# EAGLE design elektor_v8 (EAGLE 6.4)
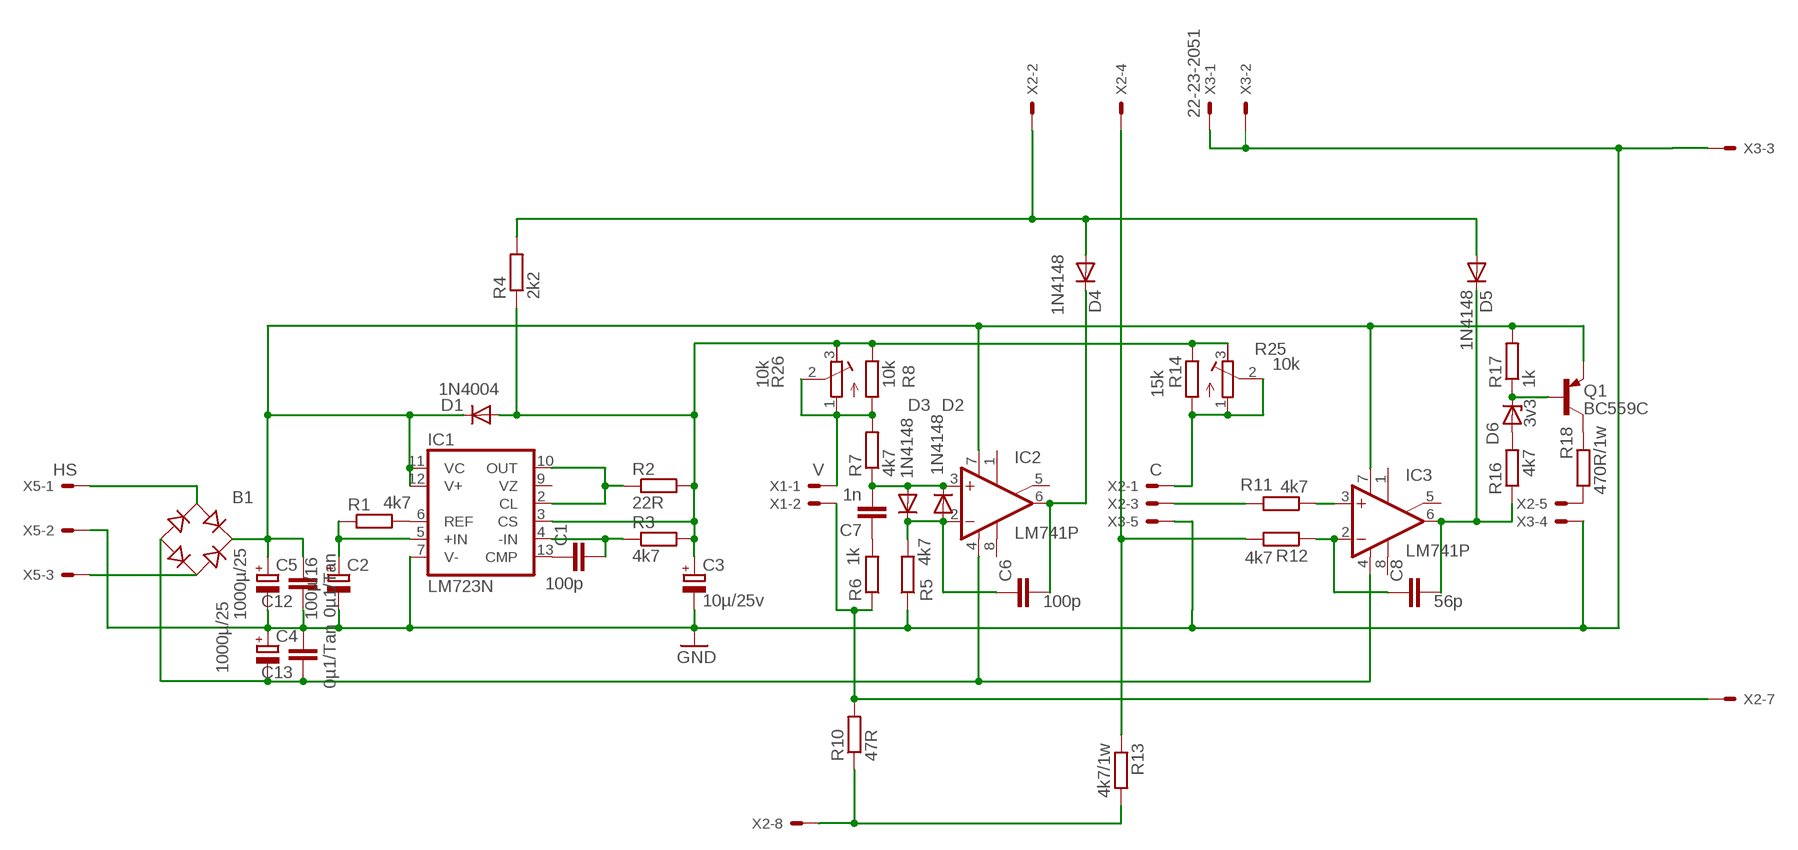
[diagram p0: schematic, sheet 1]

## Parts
B1  RB1A  [RB1A]
C1  100p  C-EU025-024X044  [C025-024X044]
C2  100µ/16  CPOL-EUE2.5-6  [E2,5-6]
C3  10µ/25v  CPOL-EUE2.5-6  [E2,5-6]
C4  1000µ/25  CPOL-EUE5-13  [E5-13]
C5  1000µ/25  CPOL-EUE5-13  [E5-13]
C6  100p  C-EU050-024X044  [C050-024X044]
C7  1n  C-EU050-024X044  [C050-024X044]
C8  56p  C-EU050-024X044  [C050-024X044]
C12  0µ1/Tan  C-EU025-024X044  [C025-024X044]
C13  0µ1/Tan  C-EU025-024X044  [C025-024X044]
D1  1N4004  [DO41-10]
D2  1N4148  1N4148DO35-7  [DO35-7]
D3  1N4148  1N4148DO35-7  [DO35-7]
D4  1N4148  1N4148DO35-7  [DO35-7]
D5  1N4148  1N4148DO35-7  [DO35-7]
D6  3v3  ZENER-DIODEDO34-7  [DO34Z7]
IC1  LM723N  [DIL14]
IC2  LM741P  [DIL08]
IC3  LM741P  [DIL08]
Q1  BC559C  [TO92-EBC]
R1  4k7  R-EU_0207/2V  [0207/2V]
R2  22R  R-EU_0207/2V  [0207/2V]
R3  4k7  R-EU_0207/2V  [0207/2V]
R4  2k2  R-EU_0204/7  [0204/7]
R5  4k7  R-EU_0207/2V  [0207/2V]
R6  1k  R-EU_0204/7  [0204/7]
R7  4k7  R-EU_0207/5V  [0207/5V]
R8  10k  R-EU_0207/2V  [0207/2V]
R10  47R  R-EU_0207/2V  [0207/2V]
R11  4k7  R-EU_0207/12  [0207/12]
R12  4k7  R-EU_0204/7  [0204/7]
R13  4k7/1w  R-EU_0204/7  [0204/7]
R14  15k  R-EU_0207/2V  [0207/2V]
R16  4k7  R-EU_0207/5V  [0207/5V]
R17  1k  R-EU_0207/5V  [0207/5V]
R18  470R/1w  R-EU_0204/7  [0204/7]
R25  10k  R-TRIMM64Y  [RTRIM64Y]
R26  10k  R-TRIMM64Y  [RTRIM64Y]
X1  V  22-23-2021  [22-23-2021]
X2  C  22-23-2081  [22-23-2081]
X3  22-23-2051  [22-23-2051]
X5  HS  22-23-2031  [22-23-2031]

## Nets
GND: C2.- C3.- C4.+ C5.- C12.1 C13.2 IC1.7(V-) R5.1 X3.1 X3.2 X3.3 X3.4 X3.5 X5.2
N$1: IC1.6(REF) R1.2
N$2: C2.+ IC1.5(+IN) R1.1
N$3: C1.1 IC1.13(CMP)
N$4: C1.2 IC1.4(-IN) R3.1
N$5: IC1.2(CL) IC1.10(OUT) R2.1
N$6: R12.2 R13.1 X2.4
N$7: C6.1 D2.A D3.C IC2.2(-IN) R5.2
N$8: R18.1 X2.5
N$9: C7.2 D2.C D3.A IC2.3(+IN) R7.1
N$10: C6.2 D4.C IC2.6(OUT)
N$11: R10.1 R13.2 X2.8
N$12: B1.AC1 X5.1
N$13: B1.AC2 X5.3
N$14: B1.+ C5.+ C12.2 D1.C IC1.11(VC) IC1.12(V+) IC2.7(V+) IC3.7(V+) Q1.E R17.2
N$15: B1.- C4.- C13.1 IC2.4(V-) IC3.4(V-)
N$16: C7.1 R6.2
N$17: R7.2 R8.1 R26.1(A) R26.2(S) X1.1
N$18: C3.+ D1.A IC1.3(CS) R2.2 R3.2 R4.1 R8.2 R14.2 R25.3(E) R26.3(E)
N$19: R6.1 R10.2 X1.2 X2.7
N$21: C8.2 D5.C IC3.6(OUT) R16.1
N$22: C8.1 IC3.2(-IN) R12.1
N$25: R11.2 X2.3
N$26: R14.1 R25.1(A) R25.2(S) X2.1
N$28: IC3.3(+IN) R11.1
N$29: D6.A R16.2
N$30: D6.C Q1.B R17.1
N$31: Q1.C R18.2
N$34: D4.A D5.A R4.2 X2.2
Unconnected: IC1.9(VZ) IC2.1(ON1) IC2.5(ON2) IC2.8(OPT) IC3.1(ON1) IC3.5(ON2) IC3.8(OPT) X2.6

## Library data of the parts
B1 = rectifier:RB1A: RECTIFIER 1 A
C1 C6-C8 C12 C13 = rcl:C-EU: CAPACITOR, European symbol
C2-C5 = rcl:CPOL-EU: POLARIZED CAPACITOR, European symbol
D1 = diode:1N4004: DIODE
D2-D5 = diode:1N4148: DIODE
D6 = diode:ZENER-DIODE: Z-Diode
IC1 = linear:*723: Positive VOLTAGE REGULATOR
IC2 IC3 = linear:*741: OP AMP
Q1 = transistor-pnp:BC559*: PNP Transistror
R1-R8 R10-R14 R16-R18 = rcl:R-EU_: RESISTOR, European symbol
R25 R26 = rcl:R-TRIMM: Trimm resistor
X1 = con-molex:22-23-2021: .100" (2.54mm) Center Header - 2 Pin; MF: MOLEX; MPN: 22-23-2021; OC_FARNELL: 1462926; OC_NEWARK: 25C3832
X2 = con-molex:22-23-2081: .100" (2.54mm) Center Header - 8 Pin; MF: MOLEX; MPN: 22-23-2081; OC_FARNELL: 1756826; OC_NEWARK: 01C7592
X3 = con-molex:22-23-2051: .100" (2.54mm) Center Header - 5 Pin; MF: MOLEX; MPN: 22-23-2051; OC_FARNELL: 1462952; OC_NEWARK: 38C9178
X5 = con-molex:22-23-2031: .100" (2.54mm) Center Header - 3 Pin; MF: MOLEX; MPN: 22-23-2031; OC_FARNELL: 1462950; OC_NEWARK: 30C0862

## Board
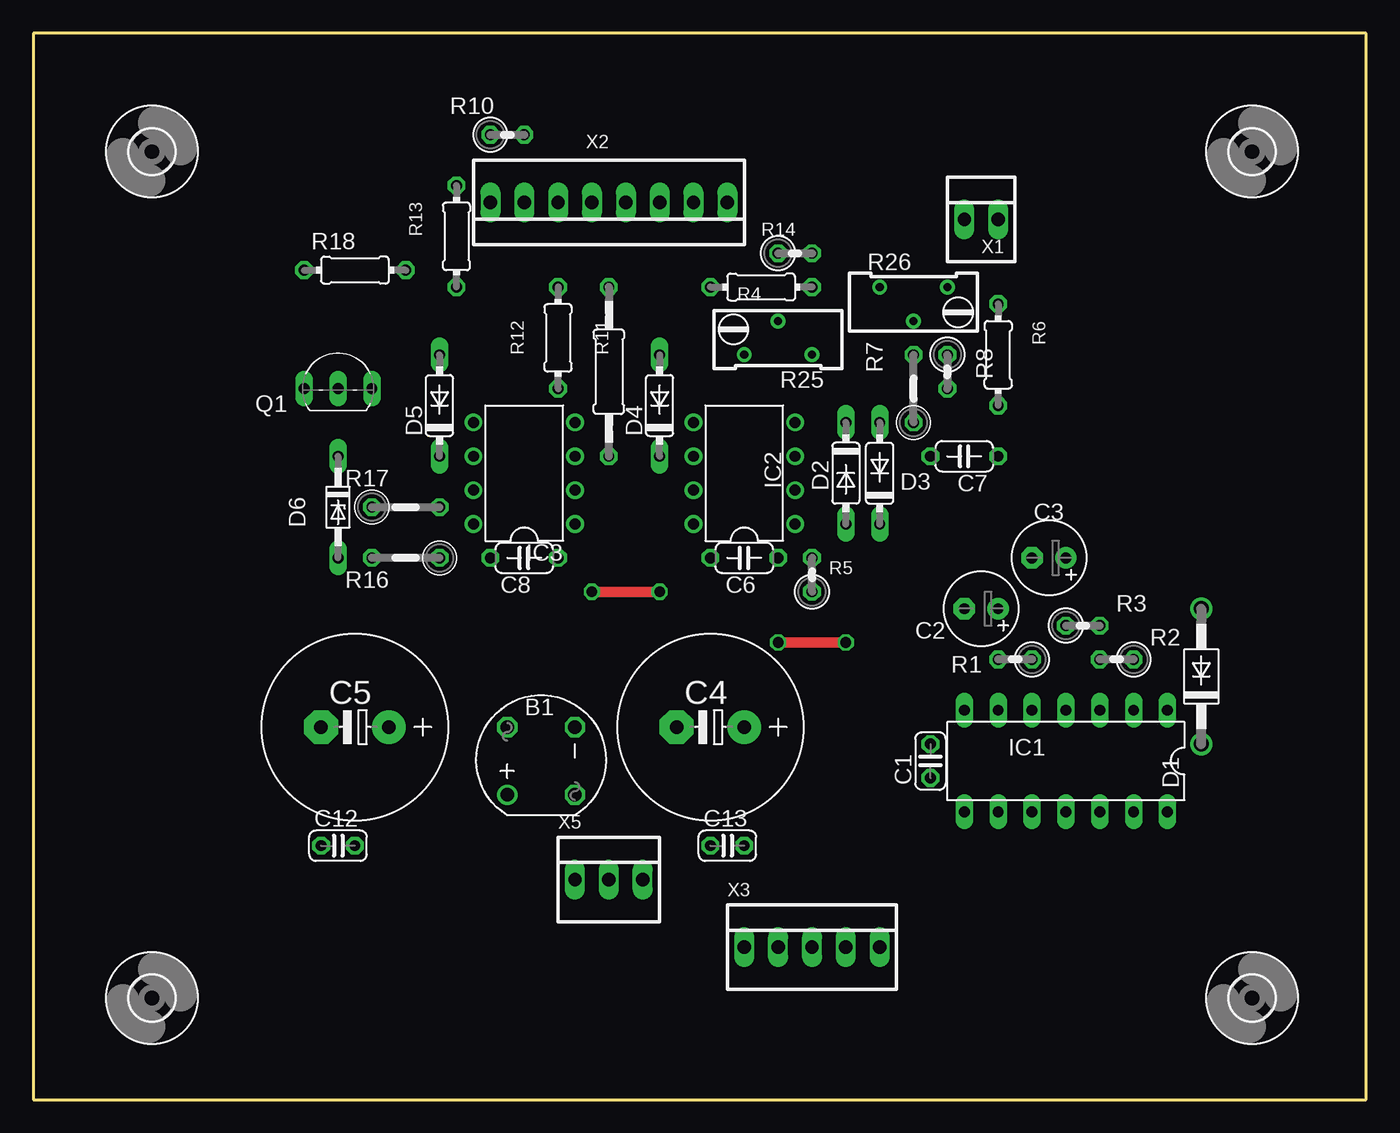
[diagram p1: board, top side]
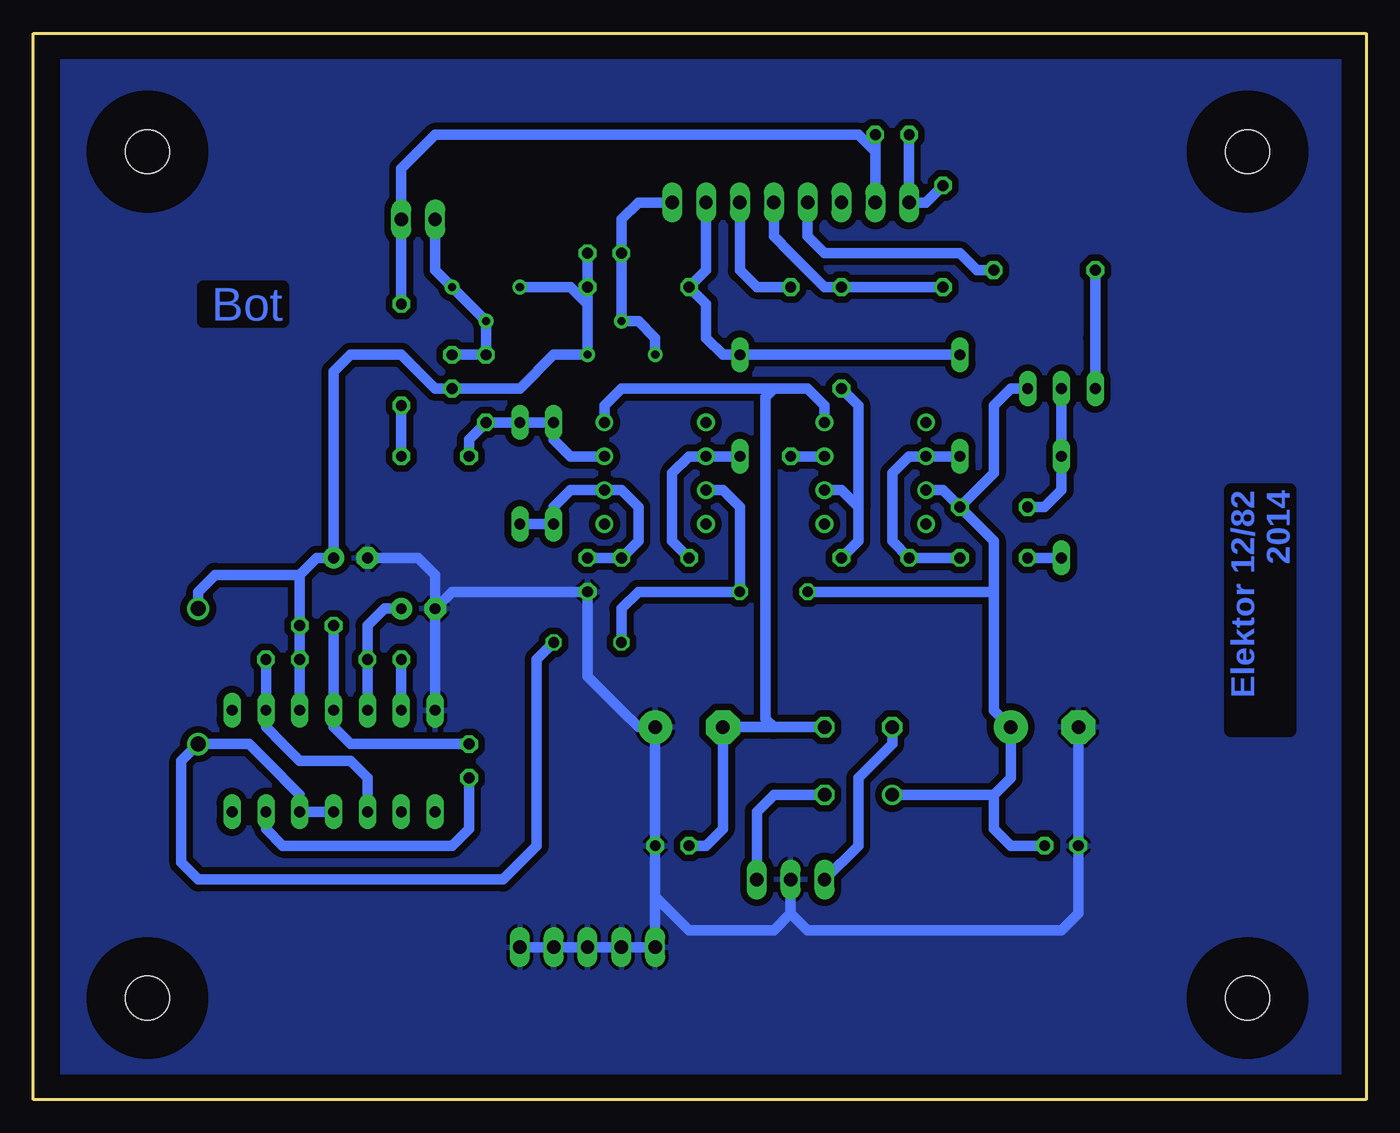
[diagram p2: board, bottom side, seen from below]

Size 100 x 80 mm. Coordinates in mm from the lower left corner, seen from the top.
Outline: 0,0 100,0 100,80 0,80 0,0
Copper layers (1*16): Top 0.035mm / dielectric 2.5mm / Bottom 0.035mm
Design rules "default *": minimum track width 12mil, minimum drill 24mil, track to track 10mil, track to pad 8mil, pad to pad 8mil, via to via 8mil, smd to smd 8mil, copper to edge 70mil, drill to drill 8mil, minimum pad ring 10mil, minimum via ring 8mil, stop-mask expansion 4mil, vias tented up to drill 0mil, thermal gap 10mil

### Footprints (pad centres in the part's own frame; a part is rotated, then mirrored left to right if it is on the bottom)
RB1A = drill 1.016: + -2.54,2.54 | drill 1.016 octagon: - 2.54,-2.54; AC1 2.54,2.54; AC2 -2.54,-2.54
C025-024X044 = drill 0.813 octagon: 1 -1.27,0; 2 1.27,0
E2,5-6 = drill 0.813 pad 1.6: + -1.27,0 | drill 0.813 pad 1.6 octagon: - 1.27,0
E5-13 = drill 1.016 pad 2.54: + -2.54,0 | drill 1.016 pad 2.54 octagon: - 2.54,0
C050-024X044 = drill 0.813 octagon: 1 -2.54,0; 2 2.54,0
DO41-10 = drill 1.118: A 5.08,0; C -5.08,0
DO35-7 = drill 0.813 long: A 3.81,0; C -3.81,0
DO34Z7 = drill 0.813 long: A 3.81,0; C -3.81,0
DIL14 = drill 0.813 long: 1 -7.62,-3.81; 2 -5.08,-3.81; 3 -2.54,-3.81; 4 0,-3.81; 5 2.54,-3.81; 6 5.08,-3.81; 7 7.62,-3.81; 8 7.62,3.81; 9 5.08,3.81; 10 2.54,3.81; 11 0,3.81; 12 -2.54,3.81; 13 -5.08,3.81; 14 -7.62,3.81
DIL08 = drill 0.813 pad 1.27: 1 -3.81,-3.81; 2 -1.27,-3.81; 3 1.27,-3.81; 4 3.81,-3.81; 5 3.81,3.81; 6 1.27,3.81; 7 -1.27,3.81; 8 -3.81,3.81
TO92-EBC = drill 0.813 long: B 0,-1.27; C -2.54,-1.27; E 2.54,-1.27
0207/2V = drill 0.813 octagon: 1 -1.27,0; 2 1.27,0
0204/7 = drill 0.813 octagon: 1 -3.81,0; 2 3.81,0
0207/5V = drill 0.813 octagon: 1 -2.54,0; 2 2.54,0
0207/12 = drill 0.813 octagon: 1 -6.35,0; 2 6.35,0
RTRIM64Y = drill 0.61: 1 0,-2.54; 2 -2.54,0; 3 0,2.54
3,3 = hole 3.3: 0,0
22-23-2021 = drill 1 long: 1 -1.27,0; 2 1.27,0
22-23-2081 = drill 1 long: 1 -8.89,0; 2 -6.35,0; 3 -3.81,0; 4 -1.27,0; 5 1.27,0; 6 3.81,0; 7 6.35,0; 8 8.89,0
22-23-2051 = drill 1 long: 1 -5.08,0; 2 -2.54,0; 3 0,0; 4 2.54,0; 5 5.08,0
22-23-2031 = drill 1 long: 1 -2.54,0; 2 0,0; 3 2.54,0

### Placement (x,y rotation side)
B1  38.1,25.4 90 top
C1  67.31,25.4 90 top
C2  71.12,36.83 180 top
C3  76.2,40.64 180 top
C4  50.8,27.94 180 top
C5  24.13,27.94 180 top
C6  53.34,40.64 180 top
C7  69.85,48.26 180 top
C8  36.83,40.64 180 top
C12  22.86,19.05 0 top
C13  52.07,19.05 0 top
D1  87.63,31.75 90 top
D2  60.96,46.99 270 top
D3  63.5,46.99 90 top
D4  46.99,52.07 90 top
D5  30.48,52.07 90 top
D6  22.86,44.45 270 top
IC1  77.47,25.4 180 top
IC2  53.34,46.99 90 top
IC3  36.83,46.99 90 top
Q1  22.86,54.61 0 top
R1  73.66,33.02 180 top
R2  81.28,33.02 180 top
R3  78.74,35.56 0 top
R4  54.61,60.96 180 top
R5  58.42,39.37 90 top
R6  72.39,55.88 270 top
R7  66.04,53.34 90 top
R8  68.58,54.61 270 top
R10  35.56,72.39 0 top
R11  43.18,54.61 90 top
R12  39.37,57.15 90 top
R13  31.75,64.77 90 top
R14  57.15,63.5 0 top
R16  27.94,40.64 180 top
R17  27.94,44.45 0 top
R18  24.13,62.23 180 top
R25  55.88,55.88 270 top
R26  66.04,60.96 90 top
U$1  [3,3]  8.89,7.62 0 top
U$2  [3,3]  91.44,7.62 0 top
U$3  [3,3]  8.89,71.12 0 top
U$4  [3,3]  91.44,71.12 0 top
X1  71.12,66.04 0 top
X2  43.18,67.31 180 top
X3  58.42,11.43 0 top
X5  43.18,16.51 0 top

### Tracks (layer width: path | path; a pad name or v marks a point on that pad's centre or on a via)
GND
  Bottom 0.8: 53.34,15.24 C13.2 C4.+ 54.61,27.94 55.88,29.21 57.15,30.48 58.42,31.75 R5.1 68.58,38.1 C2.- | 53.34,15.24 50.8,12.7 44.45,12.7 43.18,13.97 | 43.18,13.97 X5.2 | 43.18,13.97 41.91,12.7 22.86,12.7 21.59,13.97 21.59,17.78 | C5.- 21.59,17.78 | C12.1 21.59,17.78 | C3.- 71.12,40.64 69.85,39.37 C2.- | C2.- IC1.7 | 53.34,15.24 X3.1 X3.2 X3.3 X3.4 X3.5
  pour Bottom (isolate 0.5): 1.27,1.27 1.27,78.74 97.79,78.74 97.79,1.27
N$1
  Bottom 0.8: IC1.6 R1.2
N$2
  Bottom 0.8: C2.+ 73.66,36.83 74.93,35.56 R1.1 IC1.5
N$3
  Bottom 0.8: IC1.13 82.55,20.32 81.28,19.05 68.58,19.05 67.31,20.32 C1.1
N$4
  Bottom 0.8: R3.1 IC1.4 77.47,27.94 76.2,26.67 C1.2
N$5
  Bottom 0.8: R2.1 IC1.2 82.55,27.94 81.28,26.67 80.01,25.4 76.2,25.4 74.93,24.13 IC1.10
N$6
  Bottom 0.8: R13.1 R12.2 40.64,60.96 43.18,63.5 44.45,64.77 X2.4
N$7
  Bottom 0.8: D3.C D2.A 60.96,44.45 59.69,45.72 IC2.2 55.88,45.72 54.61,44.45 54.61,41.91 C6.1 R5.2
N$8
  Bottom 0.8: X2.5 41.91,64.77 40.64,63.5 30.48,63.5 29.21,62.23 R18.1
N$9
  Bottom 0.8: IC2.3 59.69,48.26 60.96,49.53 D2.C D3.A R7.1 67.31,49.53 C7.2
N$10
  Bottom 0.8: C6.2 52.07,41.91 52.07,46.99 50.8,48.26 IC2.6 D4.C
N$11
  Bottom 0.8: R13.2 33.02,67.31 X2.8 R10.1
N$12
  Bottom 0.8: X5.1 38.1,19.05 38.1,24.13 36.83,25.4 35.56,26.67 B1.AC1
N$13
  Bottom 0.8: X5.3 45.72,21.59 44.45,22.86 B1.AC2
N$14  (via drill 0.8, 0.8 pad 1.02)
  Top 0.8: v46.99,38.1 v41.91,38.1 | v55.88,34.29 v60.96,34.29
  Bottom 0.8: B1.+ 27.94,22.86 | 27.94,22.86 26.67,24.13 C5.+ 27.94,29.21 27.94,38.1 | IC3.7 31.75,45.72 R17.2 | Q1.E 26.67,53.34 27.94,52.07 27.94,46.99 29.21,45.72 R17.2 | R17.2 27.94,41.91 27.94,38.1 | IC1.11 IC1.12 80.01,22.86 82.55,25.4 83.82,26.67 D1.C 88.9,25.4 88.9,17.78 87.63,16.51 64.77,16.51 62.23,19.05 62.23,33.02 v60.96,34.29 | IC2.7 48.26,45.72 46.99,44.45 v46.99,38.1 54.61,38.1 55.88,36.83 v55.88,34.29 | v41.91,38.1 27.94,38.1 | C12.2 26.67,19.05 27.94,20.32 27.94,22.86
N$15
  Bottom 0.8: B1.- 44.45,27.94 | 44.45,27.94 C4.- 48.26,20.32 49.53,19.05 C13.1 | IC2.4 57.15,52.07 55.88,53.34 44.45,53.34 | 44.45,53.34 41.91,53.34 40.64,52.07 IC3.4 | 44.45,53.34 45.09,52.7 45.09,28.57 44.45,27.94
N$16
  Bottom 0.8: R6.2 C7.1
N$17
  Bottom 0.8: R8.1 R7.2 R26.2 R26.1 69.85,62.23 X1.1
N$18
  Bottom 0.8: 58.42,59.69 R4.1 R14.2 | 58.42,59.69 58.42,57.15 R25.3 60.96,55.88 63.5,53.34 66.04,53.34 | R26.3 59.69,60.96 58.42,59.69 | 66.04,53.34 67.31,53.34 | R8.2 67.31,53.34 | 67.31,53.34 66.04,53.34 | 67.31,53.34 R8.2 | 80.01,39.37 78.74,40.64 C3.+ 77.47,54.61 76.2,55.88 72.39,55.88 71.12,54.61 69.85,53.34 R8.2 | 80.01,39.37 R3.2 R2.2 IC1.3 | D1.A 87.63,38.1 86.36,39.37 80.01,39.37
N$19
  Bottom 0.8: R10.2 X2.7 36.83,71.12 38.1,72.39 54.61,72.39 69.85,72.39 72.39,69.85 X1.2 R6.1
N$21
  Bottom 0.8: R16.1 C8.2 35.56,41.91 35.56,46.99 34.29,48.26 IC3.6 D5.C
N$22
  Bottom 0.8: C8.1 38.1,41.91 38.1,44.45 | 38.1,44.45 39.37,45.72 IC3.2 | R12.1 38.1,52.07 38.1,44.45
N$25
  Bottom 0.8: X2.3 46.99,62.23 45.72,60.96 R11.2
N$26
  Bottom 0.8: R25.1 53.34,57.15 54.61,58.42 R25.2 R14.1 55.88,66.04 54.61,67.31 X2.1
N$28
  Bottom 0.8: R11.1 IC3.3
N$29
  Bottom 0.8: D6.A R16.2
N$30
  Bottom 0.8: Q1.B D6.C 22.86,45.72 24.13,44.45 R17.1
N$31
  Bottom 0.8: R18.2 20.32,57.15 Q1.C
N$34
  Bottom 0.8: D5.A D4.A 48.26,55.88 49.53,57.15 49.53,59.69 R4.2 49.53,62.23 X2.2

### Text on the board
Bottom: Bot | Elektor 12/82 / 2014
